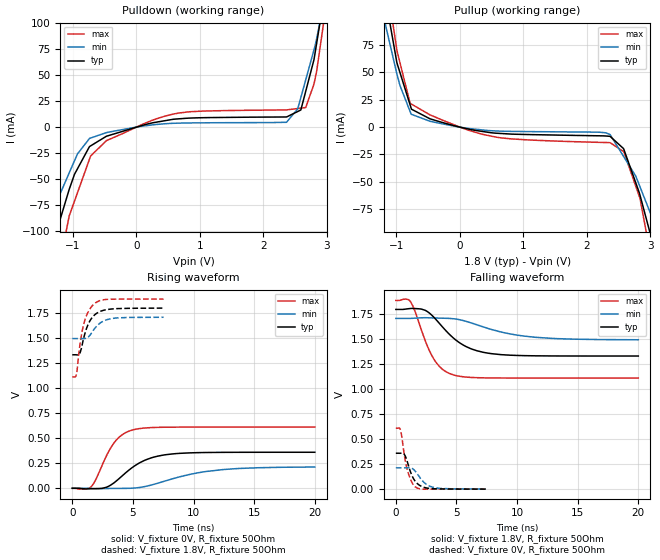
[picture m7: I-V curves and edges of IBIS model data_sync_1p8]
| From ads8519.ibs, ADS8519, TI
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|   data_sync_1p8 Model
[Model]   data_sync_1p8
Model_type   Output
Polarity   Non-Inverting
Vmeas = 0.9
Vref = 0.9
Cref = 5pF
Rref = 50
|   typ   min   max
|   (nom PVT)   (Fast PVT)   (slow PVT)
| C_comp by Frequency method (F=29Mhz)
|Average
C_comp   1.220e-11   1.118e-11   1.317e-11
|ON state: BUFFER OUTPUT TURNED HIGH
|C_comp   1.220e-11   1.118e-11   1.317e-11
|OFF state : BUFFER OUTPUT TURNED LOW
|C_comp   1.279e-11   1.160e-11   1.303e-11
| C_comp by LC Tank method (L=1nH)
| Resonant frequency (Hz)  1.67e9   1.73e9   1.61e9
|C_comp   9.092e-12   8.472e-12   9.782e-12
| Where nom  PVT is Nominal Process,  1.8V,  32C
|   Fast PVT is Strong Process,   1.89V,  -40C
|   Slow PVT is Weak Process,   1.71V,  92C
[Voltage Range]   1.8   1.71   1.89
|Ambient Temperature   25   85   -40
|Junction Temperature
[Temperature Range]   32   92   -40
[Pullup Reference]   1.8   1.71   1.89
[Pulldown Reference]   0   0   0
[Power Clamp Reference]   1.8   1.71   1.89
[GND Clamp Reference]   0   0   0
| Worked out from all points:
|   slope of the pulldown table from 0 to 0.27 V, typ, clamps not added: 62.8 ohm
|   slope of the pullup table from 0 to 0.27 V, typ, clamps not added: 83.6 ohm
|   falling waveform, V_fixture 1.8V, R_fixture 50Ohm: 20-80 % time 2.57ns typ, 4.05ns min, 1.61ns max; typ from 1.8 V to 1.33 V
|   rising waveform, V_fixture 0V, R_fixture 50Ohm: 20-80 % time 2.53ns typ, 4.39ns min, 1.62ns max; typ from 0 V to 0.36 V
|   rising waveform, V_fixture 1.8V, R_fixture 50Ohm: 20-80 % time 839ps typ, 991ps min, 733ps max; typ from 1.33 V to 1.8 V
|   falling waveform, V_fixture 0V, R_fixture 50Ohm: 20-80 % time 735ps typ, 917ps min, 600ps max; typ from 0.36 V to 0 V
[Pulldown]
|   Voltage   I(typ)   I(min)   I(max)
-1.8V     -222.2mA   -148.1mA   -316.2mA
-1.294V   -107.7mA   -77.17mA   -158.9mA
-1.058V   -59.98mA   -44.1mA    -85.52mA
-737mV    -18.62mA   -10.8mA    -30.6mA
-470.6mV  -8.721mA   -5.224mA   -12.94mA
574.6mV   7.501mA    3.675mA    12.46mA
2.365V    9.768mA    4.691mA    16.56mA
2.59V     16.49mA    28.48mA    18.27mA
2.667V    34.4mA     45.44mA    18.85mA
2.839V    80.47mA    84.77mA    53.61mA
3.007V    143.5mA    137.5mA    124.7mA
3.6V      366.9mA    323.3mA    412.4mA
[Pullup]
|   Voltage   I(typ)   I(min)   I(max)
-1.8V     357.3mA    291.5mA    437.8mA
-1.185V   122.4mA    96.78mA    144.6mA
-993.6mV  59.24mA    48.81mA    70.72mA
-784.3mV  20.33mA    14.28mA    21.77mA
-767.8mV  17.26mA    11.82mA    21.22mA
-311.4mV  4.848mA    3.444mA    7.313mA
574.6mV   -5.544mA   -3.533mA   -9.177mA
2.362V    -8.431mA   -6.672mA   -14.19mA
2.58V     -20.04mA   -27.02mA   -22.4mA
2.835V    -62.1mA    -54.52mA   -64.99mA
3.42V     -189.4mA   -140.3mA   -247.7mA
3.6V      -231.4mA   -166.7mA   -303.9mA
[Ramp]
R_load = 50
|   typ   min   max
dV/dt_r   0.215874/2.51857e-09   0.127389/4.35047e-09   0.366667/1.61459e-09
dV/dt_f   0.279982/2.5641e-09   0.128283/4.04575e-09   0.466189/1.61001e-09
[Falling Waveform]
V_fixture = 1.8V
V_fixture_min = 1.71V
V_fixture_max = 1.89V
R_fixture = 50Ohm
|   Time   V(typ)   V(min)   V(max)
0s        1.8V       1.71V      1.89V
1.185ns   1.809V     1.71V      1.881V
2.415ns   1.791V     1.717V     1.49V
3.06ns    1.731V     1.715V     1.318V
3.81ns    1.63V      1.712V     1.204V
4.695ns   1.519V     1.707V     1.146V
6.3ns     1.402V     1.662V     1.118V
8.64ns    1.348V     1.575V     1.113V
12.9ns    1.334V     1.51V      1.113V
20ns      1.333V     1.496V     1.113V
[Rising Waveform]
V_fixture = 0V
V_fixture_min = 0V
V_fixture_max = 0V
R_fixture = 50Ohm
|   Time   V(typ)   V(min)   V(max)
0s        1.676nV    2.081nV    1.371nV
1.545ns   -4.12mV    -2.493mV   14.11mV
2.79ns    9.226mV    -2.396mV   317.3mV
3.435ns   53.94mV    -1.475mV   452.2mV
4.17ns    129.8mV    -1.12mV    539.1mV
5.055ns   216.5mV    1.873mV    585mV
6.525ns   304.3mV    32.69mV    606.3mV
8.565ns   346.4mV    105mV      610.7mV
12.45ns   358.9mV    187mV      611.1mV
20ns      359.8mV    212.3mV    611.1mV
[Rising Waveform]
V_fixture = 1.8V
V_fixture_min = 1.71V
V_fixture_max = 1.89V
R_fixture = 50Ohm
|   Time   V(typ)   V(min)   V(max)
0s        1.333V     1.495V     1.113V
255ps     1.334V     1.496V     1.114V
345ps     1.333V     1.496V     1.141V
690ps     1.371V     1.495V     1.482V
1.02ns    1.536V     1.496V     1.672V
1.38ns    1.655V     1.518V     1.777V
1.8ns     1.727V     1.589V     1.841V
2.46ns    1.774V     1.663V     1.88V
3.225ns   1.791V     1.695V     1.889V
7.53ns    1.8V       1.708V     1.89V
[Falling Waveform]
V_fixture = 0V
V_fixture_min = 0V
V_fixture_max = 0V
R_fixture = 50Ohm
|   Time   V(typ)   V(min)   V(max)
0s        359.8mV    213.6mV    611.1mV
375ps     359.9mV    213.5mV    594.7mV
480ps     361.1mV    213.4mV    532.8mV
675ps     352mV      213.5mV    363.3mV
945ps     275.1mV    214.4mV    195.2mV
1.29ns    147.5mV    210.6mV    75.82mV
1.65ns    71.5mV     172.6mV    18.63mV
2.355ns   17.06mV    63.83mV    -88.6uV
3.03ns    4.7mV      19.93mV    724.7uV
7.41ns    306uV      1.31mV     9.785uV
